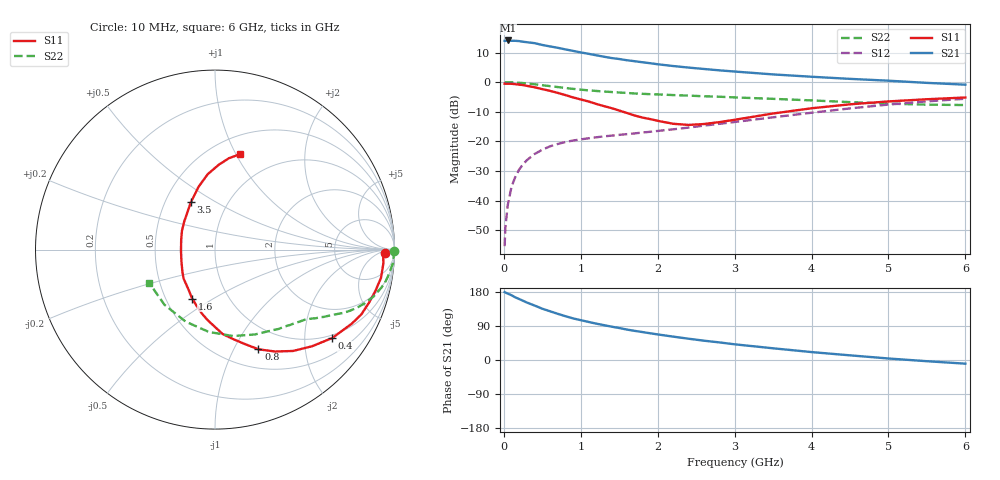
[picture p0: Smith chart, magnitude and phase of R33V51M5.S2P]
! SIEMENS Small Signal Semiconductors
! BFR181
! Si NPN RF Bipolar Junction Transistor in SOT23
! VCE = 3.5 V  IC = 1.5 mA
! Common Emitter S-Parameters:  May  1996
# GHz  S  MA  R  50
!  f  S11  S21  S12  S22
! GHz  MAG  ANG  MAG  ANG  MAG  ANG  MAG  ANG
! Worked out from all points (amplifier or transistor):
!   36 points, 10 MHz to 6 GHz, reference 50 ohm
!   highest |S21| = 14.1 dB at 50 MHz (marker M1)
!   |S21| within 3 dB of that: start of sweep to 796.1 MHz
!   unconditionally stable (mu >= 1): 1.761 GHz to 3.525 GHz
!   at 250 MHz: K = 0.19, MSG = 20.7 dB, |S12| = -27.7 dB
!   at 1.4 GHz: K = 0.87, MSG = 13.1 dB, |S12| = -18.1 dB
!   at 6 GHz: K = 0.86, MSG = 2.4 dB, |S12| = -5.6 dB
!   S11 on the Smith chart (normalised r, x): 10 MHz: 32, -11; 400 MHz: 0.91, -2.72; 800 MHz: 0.72, -1.26; 1.6 GHz: 0.68, -0.41; 3.5 GHz: 0.67, +0.39; 6 GHz: 0.68, +1.04
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0.01  0.945 -1.1  4.971 179.2  0.0017 91.2  0.997 -0.5
0.02  0.9381 -1.7  4.958 178.0  0.0035 88.2  0.9883 -0.9
0.05  0.9412 -4.8  5.058 175.3  0.0083 87.1  0.9957 -2.3
0.1  0.9383 -9.6  4.989 170.9  0.0172 83.7  0.9936 -4.5
0.15  0.9228 -14.5  4.99 165.2  0.0253 80.2  0.9835 -6.8
0.2  0.9074 -19.1  4.931 160.8  0.0336 78.2  0.9747 -8.9
0.3  0.8662 -28.5  4.723 151.6  0.0482 73.0  0.9507 -12.9
0.4  0.8183 -37.0  4.555 143.7  0.0612 68.1  0.921 -16.5
0.5  0.763 -44.9  4.245 135.3  0.0724 64.1  0.8877 -19.6
0.6  0.7128 -52.4  4.012 128.6  0.0824 60.5  0.8569 -22.1
0.8  0.6054 -66.5  3.572 115.6  0.0975 55.0  0.7983 -26.2
0.9  0.5522 -72.4  3.371 109.8  0.1034 53.2  0.7698 -27.8
1.1  0.4724 -84.8  3.013 100.5  0.1127 50.9  0.7273 -30.6
1.3  0.3947 -96.0  2.69 92.0  0.1215 49.7  0.6947 -32.8
1.6  0.3015 -115.0  2.343 80.3  0.1326 49.5  0.6575 -35.9
1.9  0.2383 -137.2  2.09 70.6  0.145 50.9  0.6269 -39.1
2.2  0.1983 -160.7  1.872 61.7  0.1598 51.9  0.6051 -42.6
2.6  0.1962 163.8  1.67 51.0  0.1843 53.4  0.5778 -47.9
3.5  0.2956 117.1  1.351 30.9  0.2549 52.8  0.5225 -64.8
4.5  0.4222 95.5  1.136 12.3  0.3604 46.0  0.46 -94.3
5.5  0.5146 81.4  0.972 -3.2  0.4734 33.6  0.4169 -132.4
6  0.551 75.1  0.906 -9.7  0.5249 26.0  0.4105 -152.8
